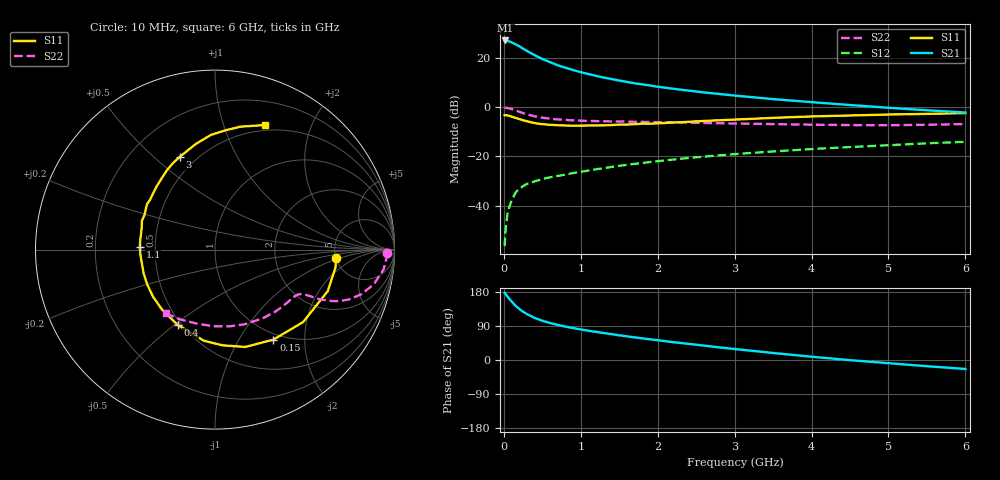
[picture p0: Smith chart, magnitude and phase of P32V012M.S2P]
! SIEMENS Small Signal Semiconductors
! BFP181
! Si NPN RF Bipolar Junction Transistor in SOT143
! VCE = 2 V  IC = 12 mA
! Common Emitter S-Parameters:  March  1996
# GHz  S  MA  R  50
!  f  S11  S21  S12  S22
! GHz  MAG  ANG  MAG  ANG  MAG  ANG  MAG  ANG
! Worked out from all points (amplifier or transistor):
!   36 points, 10 MHz to 6 GHz, reference 50 ohm
!   highest |S21| = 26.9 dB at 20 MHz (marker M1)
!   |S21| within 3 dB of that: start of sweep to 233.1 MHz
!   unconditionally stable (mu >= 1): 743 MHz to end of sweep
!   at 250 MHz: K = 0.46, MSG = 27.9 dB, |S12| = -32.1 dB
!   at 1.4 GHz: K = 1.26, MAG = 14.7 dB, |S12| = -24.4 dB
!   at 6 GHz: K = 1.06, MAG = 4.5 dB, |S12| = -14.2 dB
!   S11 on the Smith chart (normalised r, x): 10 MHz: 5.01, -0.92; 150 MHz: 0.91, -1.42; 400 MHz: 0.48, -0.51; 1.1 GHz: 0.41, +0.02; 3 GHz: 0.41, +0.61; 6 GHz: 0.44, +1.39
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0.01  0.6765 -4.2  22.13 177.3  0.0015 82.6  0.9595 -1.1
0.02  0.6785 -8.5  22.2 175.0  0.0029 79.0  0.9578 -2.6
0.05  0.6694 -20.2  21.83 166.8  0.0074 83.1  0.946 -6.7
0.1  0.6358 -39.4  20.29 154.7  0.0126 72.2  0.9044 -12.5
0.15  0.5978 -57.0  18.66 143.8  0.018 64.6  0.8501 -17.1
0.2  0.5681 -72.7  16.92 134.8  0.0221 58.9  0.7967 -20.4
0.25  0.5351 -85.4  15.13 127.4  0.0247 56.6  0.748 -22.6
0.3  0.5115 -97.0  13.65 121.4  0.0275 53.1  0.7066 -23.9
0.4  0.4687 -116.4  11.2 111.0  0.0309 50.4  0.6443 -25.4
0.5  0.4459 -131.4  9.357 103.6  0.0344 48.9  0.6036 -25.9
0.6  0.4336 -142.9  8.077 97.7  0.0374 49.0  0.5767 -26.3
0.7  0.4244 -153.1  6.98 92.6  0.0397 49.9  0.5573 -26.7
0.9  0.4145 -169.5  5.575 84.3  0.0455 49.5  0.5333 -27.7
1.1  0.4194 177.8  4.633 77.1  0.0513 50.5  0.5196 -29.3
1.3  0.4216 167.9  3.923 71.1  0.0573 50.5  0.5107 -31.5
1.6  0.4377 153.8  3.207 62.5  0.0667 51.1  0.5016 -35.1
2.2  0.4804 132.3  2.33 47.1  0.0855 49.1  0.4848 -44.0
3  0.5525 110.9  1.695 29.0  0.1102 44.2  0.46 -58.0
3.5  0.5983 100.3  1.438 18.5  0.1248 41.0  0.4478 -68.2
4.5  0.6686 84.7  1.089 -0.4  0.1531 33.2  0.4274 -91.3
5.5  0.7209 73.0  0.853 -16.4  0.1824 25.7  0.4335 -115.5
6  0.7486 68.1  0.769 -23.7  0.1961 21.5  0.4487 -127.5
